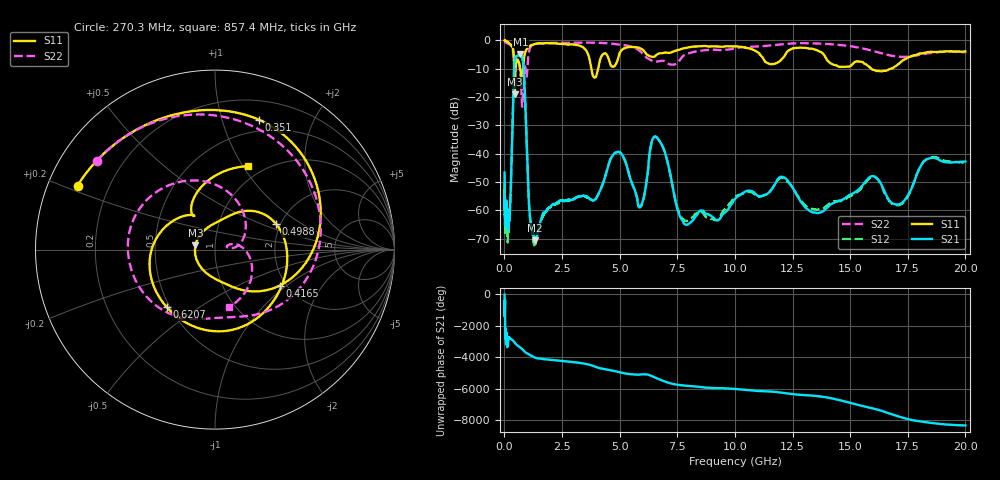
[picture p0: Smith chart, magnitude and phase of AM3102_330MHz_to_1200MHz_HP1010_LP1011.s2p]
! Date/Time: Tue, Sep 11, 2018 5:19 PM
! Network Analyzer: Agilent Technologies E8362B Rev: A.07.50.63
! Sweep from 0.010 to 20.000 GHz, 1601 Points, Sweep Type: LOG
! Power Supply: 4.949 V, 0.001 A
# Hz S DB R 50
!freq MagS11 AngS11 MagS21 AngS21 MagS12 AngS12 MagS22 AngS22
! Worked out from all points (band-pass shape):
!   1601 points, 10 MHz to 20 GHz, reference 50 ohm
!   highest |S21| = -4.79 dB at 695.6 MHz (marker M1); lowest = -70.7 dB at 1.34 GHz (marker M2)
!   |S21| within 3 dB of the highest: 437.4 MHz to 809.3 MHz (371.9 MHz wide, 59.7 % of centre)
!   lowest |S11| = -19.1 dB at 451.5 MHz (marker M3), VSWR 1.25, Z = 40.1 + j1.88 ohm
!   |S11| at or under -10 dB: 684.4 MHz to 811.7 MHz (127.3 MHz wide, 17 % of centre); 3.777 GHz to 4.069 GHz (292 MHz wide, 7.44 % of centre); 15.91 GHz to 16.77 GHz (855.7 MHz wide, 5.24 % of centre)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
!   |S22| runs from -23.4 to -0.2 dB; largest |S21 - S12| = 0.0099
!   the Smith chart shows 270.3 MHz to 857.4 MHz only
!   S11 on the Smith chart (normalised r, x): 270.3 MHz: 0.09, +0.22; 351 MHz: 0.38, +1.33; 416.5 MHz: 1.84, -0.89; 498.8 MHz: 1.89, +0.63; 620.7 MHz: 0.48, -0.37; 857.4 MHz: 0.85, +1.05
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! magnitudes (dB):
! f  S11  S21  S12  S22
! 10 MHz  0.0  -46.7  -52.7  -0.2
! 35.55 MHz  0.0  -63.3  -65.5  -0.5
! 126.4 MHz  -0.4  -63.3  -66.9  -1.0
! 270.3 MHz  -1.5  -54.7  -54.8  -1.7
! 351 MHz  -2.3  -29.8  -29.9  -3.0
! 416.5 MHz  -7.7  -11.1  -11.2  -6.2
! 447.2 MHz  -18.9  -6.9  -6.9  -8.3
! 451.5 MHz  -19.1  -6.6  -6.7  -8.4
! 498.8 MHz  -8.7  -5.7  -5.7  -7.0
! 620.7 MHz  -7.6  -5.0  -5.2  -7.3
! 695.6 MHz  -10.7  -4.8  -4.8  -11.8
! 772.3 MHz  -12.9  -5.7  -5.8  -23.4
! 857.4 MHz  -6.0  -13.3  -13.4  -9.7
! 1.087 GHz  -2.1  -60.0  -60.4  -3.3
! 1.34 GHz  -1.2  -70.7  -72.0  -1.2
! 1.59 GHz  -1.0  -63.4  -63.7  -1.0
! 3.902 GHz  -13.1  -56.4  -56.5  -0.8
! 4.878 GHz  -7.7  -39.4  -39.5  -1.4
! 5.652 GHz  -2.4  -52.7  -53.1  -2.6
! 6.58 GHz  -5.3  -34.0  -34.1  -7.5
! 7.92 GHz  -2.5  -65.1  -63.7  -4.8
! 20 GHz  -3.9  -42.8  -43.2  -4.1
